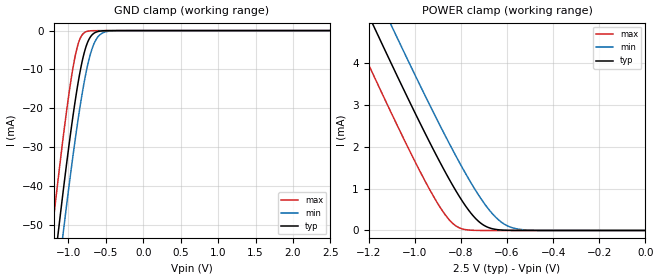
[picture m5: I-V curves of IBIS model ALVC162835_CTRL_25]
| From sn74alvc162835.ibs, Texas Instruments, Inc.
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[Model]   ALVC162835_CTRL_25
Model_type  Input
Vinl=0.7
Vinh=1.7
| variable   typ   min   max
C_comp   11.59pF   11.05pF   12.01pF
[Temperature Range]   40   100   -40
| Ambient temperature   25   85   -40
[Voltage range]   2.5   2.3   2.7
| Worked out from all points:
|   GND clamp passes 1 mA (typ) near -0.68 V on its own axis
|   POWER clamp passes 1 mA (typ) near -0.83 V on its own axis
[GND Clamp]
| ALVC162835_CTRL_25
|   Voltage   I(typ)   I(min)   I(max)
-2.5V     -300mA     -309.4mA   -288.3mA
-1.22V    -65.92mA   -76.78mA   -51.96mA
-1.15V    -54.2mA    -65.07mA   -40.19mA
-1.125V   -50.1mA    -60.96mA   -36.1mA
-1.07V    -41.27mA   -52.08mA   -27.39mA
-980mV    -27.63mA   -38.14mA   -14.46mA
-910mV    -18.08mA   -28.05mA   -6.523mA
-845mV    -10.58mA   -19.54mA   -2.069mA
-780mV    -5.041mA   -12.24mA   -440.8uA
-655mV    -630uA     -3.209mA   -15.41uA
-485mV    -21.18uA   -229.2uA   -148.8nA
2.5V      1.112nA    60.42nA    4.452pA
[POWER Clamp]
| ALVC162835_CTRL_25
|   Voltage   I(typ)   I(min)   I(max)
-2.5V     21.15mA    22.02mA    20.04mA
-1.295V   6.292mA    7.206mA    5.112mA
-1.25V    5.753mA    6.668mA    4.571mA
-1.175V   4.861mA    5.777mA    3.677mA
-1.105V   4.038mA    4.953mA    2.855mA
-1.075V   3.689mA    4.603mA    2.509mA
-945mV    2.219mA    3.118mA    1.08mA
-845mV    1.174mA    2.029mA    223.2uA
-730mV    253.2uA    906.9uA    1.947uA
-630mV    13.46uA    223.6uA    15.19nA
-515mV    218.7nA    11.36uA    63.63pA
-31.15fV  1.112nA    59.61nA    5.15pA
